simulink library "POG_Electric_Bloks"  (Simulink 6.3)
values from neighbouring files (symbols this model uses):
  al = Tipo(2)    [Flusso_Rotorico_An.m]
  bm = 0.8*N*metri*secondo/rad    (= 0.8)    [architetture_epicicloidale.m]    (also in architetture_epicicloidale_cont.m; architetture_epicicloidale_HEV.m; architetture_epicicloidale_prova.m; architetture_HEV_controllo.m)
  Iw0 = 0*wI0    [architetture_epicicloidale.m]    (also in architetture_epicicloidale_cont.m = wI0; architetture_epicicloidale_HEV.m; architetture_epicicloidale_prova.m; architetture_HEV_controllo.m)
  Jm = 1.6*kg*metri^2    (= 1.6)    [architetture_epicicloidale.m]    (also in architetture_epicicloidale_cont.m; architetture_epicicloidale_HEV.m = 1.64945909552; architetture_epicicloidale_prova.m; architetture_HEV_controllo.m = 0.529459095518)
  Li = 0.1*Henry    (= 0.1)    [architetture_epicicloidale.m]    (also in architetture_epicicloidale_cont.m; architetture_epicicloidale_HEV.m; architetture_epicicloidale_prova.m; architetture_HEV_controllo.m)
  m = 5    [architetture_epicicloidale.m]    (also in architetture_epicicloidale_cont.m; architetture_epicicloidale_HEV.m; architetture_epicicloidale_prova.m; architetture_HEV_controllo.m)
  Mi = 0.08*Henry    (= 0.08)    [architetture_epicicloidale.m]    (also in architetture_epicicloidale_cont.m; architetture_epicicloidale_HEV.m; architetture_epicicloidale_prova.m; architetture_HEV_controllo.m)
  ms = 0.001*secondo    (= 0.001)    [architetture_epicicloidale.m]    (also in architetture_epicicloidale_cont.m; architetture_epicicloidale_HEV.m; architetture_epicicloidale_prova.m; architetture_HEV_controllo.m)
  Nar = 200    [architetture_epicicloidale.m]    (also in architetture_epicicloidale_cont.m; architetture_epicicloidale_HEV.m; architetture_epicicloidale_prova.m; architetture_HEV_controllo.m)
  Nc = 30    [architetture_epicicloidale.m]    (also in architetture_epicicloidale_cont.m; architetture_epicicloidale_HEV.m; architetture_epicicloidale_prova.m; architetture_HEV_controllo.m)
  p = 1    [architetture_epicicloidale.m]    (also in architetture_epicicloidale_cont.m; architetture_epicicloidale_HEV.m; architetture_epicicloidale_prova.m; architetture_HEV_controllo.m)
  Phir = 0.02*Weber    (= 0.02)    [architetture_epicicloidale.m]    (also in architetture_epicicloidale_cont.m; architetture_epicicloidale_HEV.m; architetture_epicicloidale_prova.m; architetture_HEV_controllo.m)
  Ri = 3*Ohm    (= 3)    [architetture_epicicloidale.m]    (also in architetture_epicicloidale_cont.m; architetture_epicicloidale_HEV.m; architetture_epicicloidale_prova.m; architetture_HEV_controllo.m = 0.1)
  Rr = 0.905*m    (= 0.905)    [CVT_New.m]    (also in CVT_New_th.m)
  Star = Si    [architetture_epicicloidale.m]    (also in architetture_epicicloidale_cont.m; architetture_epicicloidale_HEV.m; architetture_epicicloidale_prova.m; architetture_HEV_controllo.m)
  Thm0 = 0    [architetture_epicicloidale.m]    (also in architetture_epicicloidale_cont.m; architetture_epicicloidale_HEV.m; architetture_epicicloidale_prova.m; architetture_HEV_controllo.m)
  Tipo = eval(Flusso(ij).Tipo)    [architetture_epicicloidale.m]    (also in architetture_epicicloidale_cont.m; architetture_epicicloidale_HEV.m; architetture_epicicloidale_prova.m; architetture_HEV_controllo.m)
  Wm0 = 0*Wr_d    (= 0)    [architetture_epicicloidale.m]    (also in architetture_epicicloidale_cont.m = 62.5; architetture_epicicloidale_HEV.m; architetture_epicicloidale_prova.m; architetture_HEV_controllo.m)
undefined symbols (not defined in the file or in its folder): Ib0, Lr, Ls, Lwe, mr, Mr0, Ms0, Msr0, Rs, Rwe
libraries: simulink x10
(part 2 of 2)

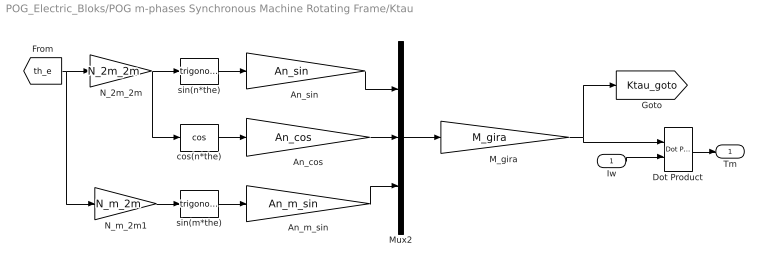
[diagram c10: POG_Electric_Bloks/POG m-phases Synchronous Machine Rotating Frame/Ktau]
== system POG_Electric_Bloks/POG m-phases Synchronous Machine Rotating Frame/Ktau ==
  Iw : Inport
  An_cos : Gain  Gain=An_cos  Multiplication=Matrix(K*u) (u vector)
  An_m_sin : Gain  Gain=An_m_sin  Multiplication=Matrix(K*u) (u vector)
  "An_sin " : Gain  Gain=An_sin  Multiplication=Matrix(K*u) (u vector)
  Dot Product : simulink/Math Operations/Dot Product  InputSameDT=on  OutDataType=sfix(16)  OutScaling=2^-10  DoSatur=off
  "M_gira " : Gain  Gain=M_gira  Multiplication=Matrix(K*u) (u vector)
  Mux2 : Mux  Inputs=3
  N_2m_2m : Gain  Gain=N_2m_2m  Multiplication=Matrix(K*u) (u vector)
  N_m_2m1 : Gain  Gain=N_m_2m  Multiplication=Matrix(K*u) (u vector)
  cos(n*the) : Trigonometry  Operator=cos
  sin(m*the) : Trigonometry
  sin(n*the) : Trigonometry
  Tm : Outport
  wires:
  An_m_sin/1 -> Mux2/3
  "M_gira "/1 -> [Ktau_goto], Dot Product/1
  Mux2/1 -> "M_gira "/1
  An_cos/1 -> Mux2/2
  "An_sin "/1 -> Mux2/1
  sin(m*the)/1 -> An_m_sin/1
  N_m_2m1/1 -> sin(m*the)/1
  cos(n*the)/1 -> An_cos/1
  sin(n*the)/1 -> "An_sin "/1
  N_2m_2m/1 -> cos(n*the)/1, sin(n*the)/1
  [th_e] -> N_m_2m1/1, N_2m_2m/1
  Iw/1 -> Dot Product/2
  Dot Product/1 -> Tm/1

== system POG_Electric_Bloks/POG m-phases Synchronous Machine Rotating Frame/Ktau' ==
  Wm : Inport
  Product : Product  Multiplication=Matrix(*)
  Ew : Outport
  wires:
  [Ktau_goto] -> Product/1
  Product/1 -> Ew/1
  Wm/1 -> Product/2

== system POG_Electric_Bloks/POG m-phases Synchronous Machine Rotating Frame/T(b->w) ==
  Vt : Inport
  Product : Product  Multiplication=Matrix(*)
  Vw : Outport
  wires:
  [T_w_b] -> Product/1
  Product/1 -> Vw/1
  Vt/1 -> Product/2

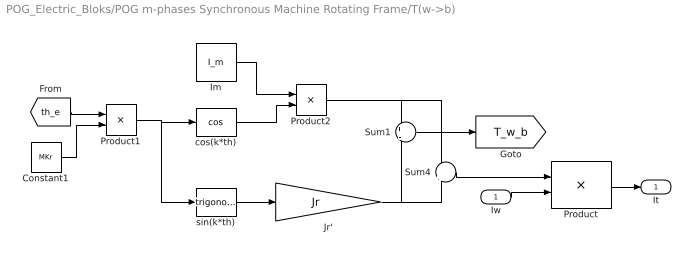
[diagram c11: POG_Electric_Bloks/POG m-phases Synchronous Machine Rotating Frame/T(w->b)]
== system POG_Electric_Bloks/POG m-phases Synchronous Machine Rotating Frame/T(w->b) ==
  Iw : Inport
  Constant1 : Constant  Value=MKr
  Im : Constant  Value=I_m  VectorParams1D=off
  Jr' : Gain  Gain=Jr  Multiplication=Matrix(K*u)
  Product : Product  Multiplication=Matrix(*)
  Product1 : Product
  Product2 : Product
  Sum1 : Sum  Inputs=+|-
  Sum4 : Sum  Inputs=+|+
  cos(k*th) : Trigonometry  Operator=cos
  sin(k*th) : Trigonometry
  It : Outport
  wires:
  Sum1/1 -> [T_w_b]
  sin(k*th)/1 -> Jr'/1
  [th_e] -> Product1/1
  Constant1/1 -> Product1/2
  Product1/1 -> cos(k*th)/1, sin(k*th)/1
  cos(k*th)/1 -> Product2/2
  Im/1 -> Product2/1
  Product2/1 -> Sum1/1, Sum4/1
  Jr'/1 -> Sum1/2, Sum4/2
  Iw/1 -> Product/2
  Product/1 -> It/1
  Sum4/1 -> Product/1

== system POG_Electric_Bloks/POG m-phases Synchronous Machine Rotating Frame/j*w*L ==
  In1 : Inport
  Gain1 : Gain  Gain=Kr  Multiplication=Matrix(K*u) (u vector)
  Gain2 : Gain  Gain=Jr  Multiplication=Matrix(K*u) (u vector)
  Gain4 : Gain  Gain=MLb  Multiplication=Matrix(K*u) (u vector)
  Product : Product
  Out1 : Outport
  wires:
  Gain2/1 -> Out1/1
  Product/1 -> Gain2/1
  Gain4/1 -> Product/2
  Gain1/1 -> Product/1
  [w_e] -> Gain1/1
  In1/1 -> Gain4/1
